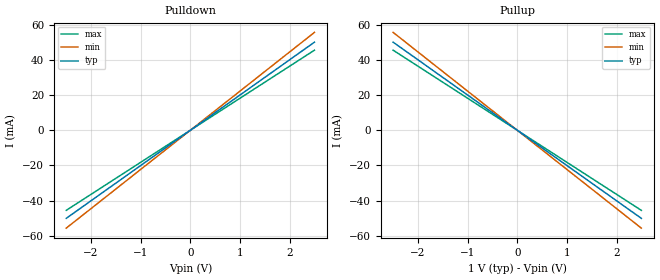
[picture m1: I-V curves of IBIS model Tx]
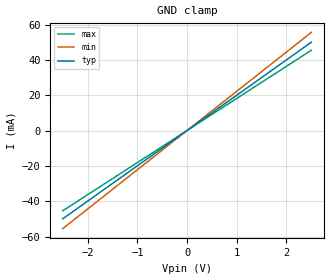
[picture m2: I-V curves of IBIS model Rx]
[IBIS Ver]   5.0
[Disclaimer]   This IBIS file has been created by Mentor Graphics
[File Name]   legacy_bird125.ibs
[File Rev]   1.0
[Date]   September 3, 2012
[Source]   Mentor Graphics
[Notes]   This IBIS file is an illustration for package and on-die
   interconnect modeling using the concepts proposed in
   BIRD 116, 118, 125 and 145.
[Copyright]   No Copyright
[Component]   legacy
[Manufacturer]  No Manufacturer
[Package]
R_pkg 0.001m   NA   NA
L_pkg 0.001nH  NA   NA
C_pkg 0.001pF  NA   NA
[Package Model]  A_12_pin_pkg_model
[Pin]  signal_name   model_name   R_pin  L_pin  C_pin
AW10 RX[0]_N MODELCALL NA NA NA | Diff_Package pkg_{Corner}.mod pkg_{Corner} Length=0.01755
AV10 RX[0]_P MODELCALL NA NA NA | Diff_Package pkg_{Corner}.mod pkg_{Corner} Length=0.01755
AW13 RX[1]_N MODELCALL NA NA NA | Diff_Package pkg_{Corner}.mod pkg_{Corner} Length=0.01565
AV13 RX[1]_P MODELCALL NA NA NA | Diff_Package pkg_{Corner}.mod pkg_{Corner} Length=0.01565
AW8 RX[10]_N MODELCALL NA NA NA | Diff_Package pkg_{Corner}.mod pkg_{Corner} Length=0.01785
AV8 RX[10]_P MODELCALL NA NA NA | Diff_Package pkg_{Corner}.mod pkg_{Corner} Length=0.01785
AR10 TX[0]_N MODELCALL NA NA NA | Diff_Package pkg_{Corner}.mod pkg_{Corner} Length=0.01375
AP10 TX[0]_P MODELCALL NA NA NA | Diff_Package pkg_{Corner}.mod pkg_{Corner} Length=0.01375
AR13 TX[1]_N MODELCALL NA NA NA | Diff_Package pkg_{Corner}.mod pkg_{Corner} Length=0.01165
AP13 TX[1]_P MODELCALL NA NA NA | Diff_Package pkg_{Corner}.mod pkg_{Corner} Length=0.01165
AR8 TX[10]_N MODELCALL NA NA NA | Diff_Package pkg_{Corner}.mod pkg_{Corner} Length=0.01340
AP8 TX[10]_P MODELCALL NA NA NA | Diff_Package pkg_{Corner}.mod pkg_{Corner} Length=0.01340
[Diff_Pin]  inv_pin  vdiff  tdelay_typ  tdelay_min  tdelay_max
AV10   AW10   0.1V   0.0ns   0.0ns   0.0ns
AV13   AW13   0.1V   0.0ns   0.0ns   0.0ns
AV8   AW8   0.1V   0.0ns   0.0ns   0.0ns
AP10   AR10   0.1V   0.0ns   0.0ns   0.0ns
AP13   AR13   0.1V   0.0ns   0.0ns   0.0ns
AP8   AR8   0.1V   0.0ns   0.0ns   0.0ns
[Node Declarations]
TxAsignal_P  TxAsignal_N   | List of Tx die nodes
RxAsignal_P  RxAsignal_N   | List of Rx die nodes
TxPad_P   TxPad_N   | List of Tx die pads
RxPad_P   RxPad_N   | List of Rx die pads
[End Node Declarations]
[Model Call] Tx   | Instantiates [Model] named "Tx"
Diff_Signal_pin  AR10  AP10   | This subparameter will need a BIRD to
Diff_Signal_pin  AR13  AP13   | allow for more than just one occurence
Diff_Signal_pin  AR8   AP8
Port_map   A_signal_pos   TxAsignal_P  | Connection to explicit die-node
Port_map   A_signal_neg   TxAsignal_N  | Connection to explicit die-node
[End Model Call]
[Model Call] Rx   | Instantiates [Model] named "Rx"
Diff_Signal_pin  AW10  AV10   | This subparameter will need a BIRD to
Diff_Signal_pin  AW13  AV13   | allow for more than just one occurence
Diff_Signal_pin  AW8   AV8
Port_map   A_signal_pos   RxAsignal_P  | Connection to explicit die-node
Port_map   A_signal_neg   RxAsignal_N  | Connection to explicit die-node
[End Model Call]
[Circuit Call] On_Die_Tx   | Instantiates [External Circuit] named "On_Die_Tx"
Port_map  dieP  TxAsignal_P  | Port to explicit Tx [Model] terminal connection
Port_map  dieN  TxAsignal_N  | Port to explicit Tx [Model] terminal connection
Port_map  padP  TxPad_P   | Port to explicit Tx die pad connection
Port_map  padN  TxPad_N   | Port to explicit Tx die pad connection
[End Circuit Call]
[Circuit Call] On_Die_Rx   | Instantiates [External Circuit] named "On_Die_Rx"
Port_map  dieP  RxAsignal_P  | Port to explicit Rx [Model] terminal connection
Port_map  dieN  RxAsignal_N  | Port to explicit Rx [Model] terminal connection
Port_map  padP  RxPad_P   | Port to explicit Rx die pad connection
Port_map  padN  RxPad_N   | Port to explicit Rx die pad connection
[End Circuit Call]
[External Circuit] On_Die_Tx
Language IBIS-ISS
| Corner corner_name file_name .subckt name
Corner  Typ  On_Die.iss  On_Die
Corner  Min  On_Die.iss  On_Die
Corner  Max  On_Die.iss  On_Die
Parameters  TSFile = thisfile.ibs(TreeRootName(Tx_TSFile)) "Tx_typ.s4p"
| Ports are in same order as defined in IBIS-ISS
Ports  dieP  dieN  padP  padM
[End External Circuit]
[External Circuit] On_Die_Rx
Language IBIS-ISS
| Corner corner_name file_name .subckt name
Corner  Typ  On_Die.iss  On_Die
Corner  Min  On_Die.iss  On_Die
Corner  Max  On_Die.iss  On_Die
Parameters  TSFile = thisfile.ibs(TreeRootName(Rx_TSFile)) "Rx_typ.s4p"
| Ports are in same order as defined in IBIS-ISS
Ports  dieP  dieN  padP  padM
[End External Circuit]
|   PACKAGE  MODEL
[Define Package Model]  A_12_pin_pkg_model
[Manufacturer]   Noname Company, Inc.
[OEM]   Another Noname Package Company, Inc.
[Description]   12-pin illustration package model
[Number Of Pins]  12
[Pin Numbers]
AW10
AV10
AW13
AV13
AW8
AV8
AR10
AP10
AR13
AP13
AR8
AP8
[Package Circuit]
Port_map  PortMapName_1  Position = thisfile.ibs(TreeRootName(PinPosition))  1
pins  AW10  AW13  AW8  AR10  AR13  AR8
Port_map  PortMapName_2  Position = thisfile.ibs(TreeRootName(PinPosition))  1
pins  AV10  AV13  AV8  AP10  AP13  AP8
Port_map  PortMapName_3  Position = thisfile.ibs(TreeRootName(PadPosition))  1
nodes  RxPadP  TxPadP
Port_map  PortMapName_4  Position = thisfile.ibs(TreeRootName(PadPosition))  1
nodes  RxPadN  TxPadN
| On the above lines, the Parameter Tree is assumed to have a Dependency Table
| such that when "PinPosition" has values of 1-3, "PadPosition" is assigned 1,
| and when "PinPosition" has values of 4-5, "PadPosition" is assigned 2.
Language IBIS-ISS
| Corner  corner_name  file_name  .subckt name
Corner  Typ  PackageModel.iss  Pkg_Model
Corner  Min  PackageModel.iss  Pkg_Model
Corner  Max  PackageModel.iss  Pkg_Model
Parameters  RLGCmodelName = thisfile.ibs(TreeRootName(RLGCmodelName)) "rlgc_typ"
Parameters  Length = thisfile.ibs(TreeRootName(Length)) 0.017
| Ports are in same order as defined in IBIS-ISS
Ports  PortMapName_3  PortMapName_4  PortMapName_1  PortMapName_2
[End Package Circuit]
[End Package Model]
| Models and submodels in the file (2): Tx (Output), Rx (Input)
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|   MODEL Tx
[Model] Tx
Model_type Output
C_comp 0.5p 0.5p 0.5p
Cref = 0
Vref = 0.5
Rref = 50
Vmeas = 0.5
[Temperature_Range] 25 100 0
[Voltage Range] 1.0 1.0 1.0
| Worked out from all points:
|   slope of the pulldown table from 0 to 0.15 V, typ, clamps not added: 50 ohm
|   slope of the pullup table from 0 to 0.15 V, typ, clamps not added: 50 ohm
| On-Die Tstonefile Tx_typ.s4p Tx_min.s4p Tx_max.s4p
| Diff_Package pkg_{Corner}.mod pkg_{Corner} Length=0.02
| Diff_Package_Coupled pkg_cpl_{Corner}.mod pkg_cpl_{Corner} Length=0.02
[Pulldown]
-2.5V     -50mA      -55.56mA   -45.45mA
0V        0A         0A         0A
2.5V      50mA       55.56mA    45.45mA
[Pullup]
-2.5V     50mA       55.56mA    45.45mA
0V        0A         0A         0A
2.5V      -50mA      -55.56mA   -45.45mA
[Ramp]
dV/dt_r 0.3/60p 0.3/60p 0.3/60p
dV/dt_f 0.3/60p 0.3/60p 0.3/60p
|   MODEL Rx
[Model] Rx
Model_type Input
C_comp 0.5p 0.5p 0.5p
Vinh = 0.55
Vinl = 0.45
[Temperature_Range] 25 100 0
[Voltage Range] 1.0 1.0 1.0
| On-Die Tstonefile Rx_typ.s4p Rx_min.s4p Rx_max.s4p
| Diff_Package pkg_{Corner}.mod pkg_{Corner} Length=0.01
| Diff_Package_Coupled pkg_cpl_{Corner}.mod pkg_cpl_{Corner} Length=0.01
[GND Clamp]
-2.5V     -50mA      -55.56mA   -45.45mA
0V        0A         0A         0A
2.5V      50mA       55.56mA    45.45mA
